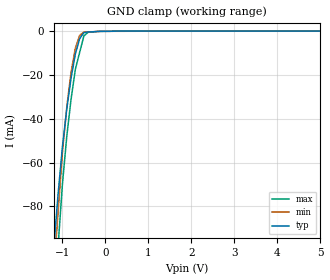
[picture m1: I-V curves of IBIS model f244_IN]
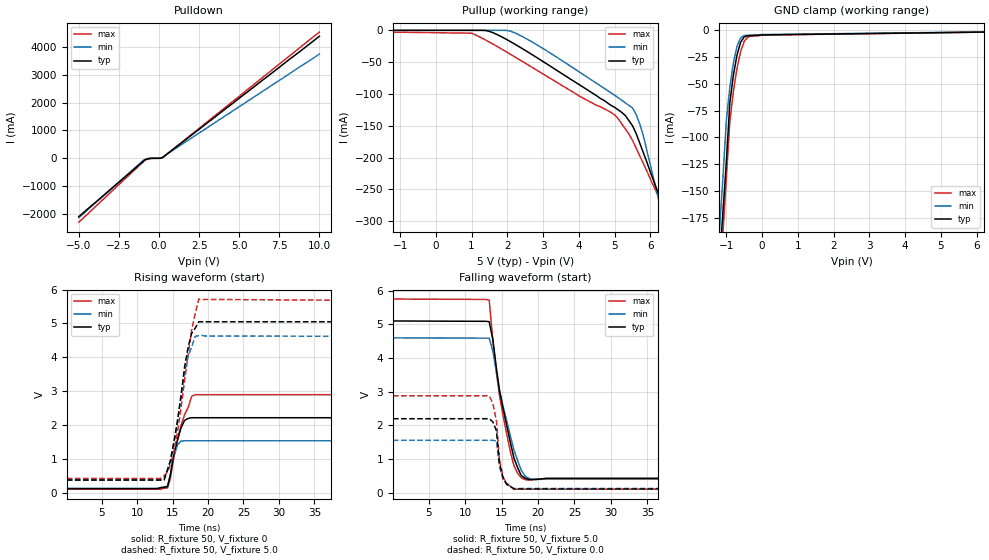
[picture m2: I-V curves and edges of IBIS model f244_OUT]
| TEXAS INSTRUMENTS INCORPORATED
| Standard Linear and Logic Group
| IBIS Model of SN74F244
| OCTAL BUFFERS/DRIVERS WITH 3-STATE OUTPUTS
| SOIC 20-pin (DW), SOP 20-pin (NS), SSOP 20-pin (DB), PDIP 20-pin (N)
[IBIS Ver]   3.2
[Comment Char]  |_char
[File Name]   sn74f244.ibs
[File Rev]   2.1 I_die
[Date]   Nov. 04, 2004
[Source]   File originated at Texas Instruments, Inc.
[Notes]   The following is a sample IBIS file for the F244.
   - FILE REV HISTORY
   - 2.1 Re-Release IBIS file on 11/05/04
   - Power-clamp data deleted as there is no power-clamp diode.
|   - All test data contained in this file are derived from
|   actual measurements.
|   - File created by Nobuhisa Ohtsubo, SLL Product Engineering.
[Disclaimer] Property of Texas Instruments Incorporated.  Unauthorized
   reproduction and/or distribution is strictly prohibited.
   This product is protected under copyright law.
   Created 2000, (C) Copyright 2000, Texas Instruments Inc.,
   All Rights Reserved.
   UNLESS THERE IS A SIGNED, WRITTEN AGREEMENT TO THE
   CONTRARY, TEXAS INSTRUMENTS () IS PROVIDING THE IBIS
   MODELS  AND WITHOUT ANY WARRANTY, EXPRESSED OR
   IMPLIED.  TI assumes no liability for:
   1) the accuracy of the IBIS models provided to your
   company;
   2) the proper functioning of these IBIS Models in your
   design or for any resulting applications; or
   3) infringement of patents, copyrights or intellectual
   property rights resulting from your use of these IBIS
   models.
   TI provides IBIS Models as a service to our customers.
   You and your company shall not distribute, sell or give
   these models to anyone else without prior written
   permission from TI.
   TI reserves the right to make changes to our products or
   to discontinue any semiconductor product or service
   without notice, and advises our customers to obtain the
   latest version of relevant information to verify, before
   placing orders, that the information being relied on is
   current.
   Please be aware that your receipt and use of the IBIS
   information provided shall serve as acceptance of these
   terms and conditions.  If you do not accept these terms,
   you should return or destroy the IBIS models and any
   other accompanying information immediately.
|   Component F244_DW
[Component]   f244_DW
[Manufacturer]  Texas Instruments, Inc.
[Package]
|   typ   min   max
R_pkg   0.038   0.033   0.045
L_pkg   5.012nH   4.110nH   6.349nH
C_pkg   0.717pF   0.530pF   0.868pF
[Pin]   signal_name   model_name   R_pin   L_pin   C_pin
1   1OE_NOT   f244_IN   0.058   5.115nH   0.725pF
2   1A1   f244_IN   0.053   4.591nH   0.724pF
3   2Y4   f244_OUT   0.049   3.754nH   0.572pF
4   1A2   f244_IN   0.029   2.549nH   0.388pF
5   2Y3   f244_OUT   0.031   2.317nH   0.316pF
6   1A3   f244_IN   0.031   2.317nH   0.316pF
7   2Y2   f244_OUT   0.029   2.556nH   0.399pF
8   1A4   f244_IN   0.049   3.754nH   0.579pF
9   2Y1   f244_OUT   0.053   4.591nH   0.724pF
10   GND   GND   0.058   5.115nH   0.725pF
11   2A1   f244_IN   0.058   5.115nH   0.725pF
12   1Y4   f244_OUT   0.053   4.591nH   0.724pF
13   2A2   f244_IN   0.049   3.754nH   0.579pF
14   1Y3   f244_OUT   0.029   2.557nH   0.399pF
15   2A3   f244_IN   0.031   2.317nH   0.316pF
16   1Y2   f244_OUT   0.031   2.317nH   0.316pF
17   2A4   f244_IN   0.029   2.557nH   0.399pF
18   1Y1   f244_OUT   0.049   3.754nH   0.579pF
19   2OE_NOT   f244_IN   0.053   4.591nH   0.724pF
20   VCC   POWER   0.058   5.115nH   0.725pF
|   Component F244_NS
[Component]   f244_NS
[Manufacturer]  Texas Instruments, Inc.
[Package]
|   typ   min   max
R_pkg   0.044   0.029   0.058
L_pkg   3.666nH   2.317nH   5.115nH
C_pkg   0.548pF   0.316pF   0.725pF
[Pin]   signal_name   model_name   R_pin   L_pin   C_pin
1   1OE_NOT   f244_IN   0.058   5.115nH   0.725pF
2   1A1   f244_IN   0.053   4.591nH   0.724pF
3   2Y4   f244_OUT   0.049   3.754nH   0.572pF
4   1A2   f244_IN   0.029   2.549nH   0.388pF
5   2Y3   f244_OUT   0.031   2.317nH   0.316pF
6   1A3   f244_IN   0.031   2.317nH   0.316pF
7   2Y2   f244_OUT   0.029   2.556nH   0.399pF
8   1A4   f244_IN   0.049   3.754nH   0.579pF
9   2Y1   f244_OUT   0.053   4.591nH   0.724pF
10   GND   GND   0.058   5.115nH   0.725pF
11   2A1   f244_IN   0.058   5.115nH   0.725pF
12   1Y4   f244_OUT   0.053   4.591nH   0.724pF
13   2A2   f244_IN   0.049   3.754nH   0.579pF
14   1Y3   f244_OUT   0.029   2.557nH   0.399pF
15   2A3   f244_IN   0.031   2.317nH   0.316pF
16   1Y2   f244_OUT   0.031   2.317nH   0.316pF
17   2A4   f244_IN   0.029   2.557nH   0.399pF
18   1Y1   f244_OUT   0.049   3.754nH   0.579pF
19   2OE_NOT   f244_IN   0.053   4.591nH   0.724pF
20   VCC   POWER   0.058   5.115nH   0.725pF
|   Component F244_DB
[Component]   f244_DB
[Manufacturer]  Texas Instruments, Inc.
[Package]
|   typ   min   max
R_pkg   0.040   0.035   0.051
L_pkg   3.495nH   3.035nH   4.314nH
C_pkg   0.420pF   0.346pF   0.502pF
[Pin]   signal_name   model_name   R_pin   L_pin   C_pin
1   1OE_NOT   f244_IN   0.049   4.310nH   0.502pF
2   1A1   f244_IN   0.048   3.903nH   0.487pF
3   2Y4   f244_OUT   0.035   3.189nH   0.396pF
4   1A2   f244_IN   0.035   3.036nH   0.347pF
5   2Y3   f244_OUT   0.035   3.035nH   0.367pF
6   1A3   f244_IN   0.035   3.035nH   0.367pF
7   2Y2   f244_OUT   0.035   3.036nH   0.347pF
8   1A4   f244_IN   0.035   3.189nH   0.397pF
9   2Y1   f244_OUT   0.047   3.899nH   0.488pF
10   GND   GND   0.051   4.314nH   0.500pF
11   2A1   f244_IN   0.051   4.314nH   0.500pF
12   1Y4   f244_OUT   0.047   3.899nH   0.488pF
13   2A2   f244_IN   0.035   3.189nH   0.397pF
14   1Y3   f244_OUT   0.035   3.036nH   0.346pF
15   2A3   f244_IN   0.035   3.035nH   0.367pF
16   1Y2   f244_OUT   0.035   3.035nH   0.367pF
17   2A4   f244_IN   0.035   3.036nH   0.346pF
18   1Y1   f244_OUT   0.035   3.189nH   0.397pF
19   2OE_NOT   f244_IN   0.047   3.899nH   0.488pF
20   VCC   POWER   0.051   4.314nH   0.502pF
|   Component F244_N
[Component]   f244_N
[Manufacturer]   Texas Instruments, Inc.
[Package]
|   typ   min   max
R_pkg   4.300e-02   3.800e-02   5.000e-02
L_pkg   7.384e-09   4.680e-09   1.032e-08
C_pkg   5.100e-13   2.310e-13   8.210e-13
[PIN]   signal_name   model_name   R_pin   L_pin   C_pin
1   1OE_NOT   f244_IN   4.200e-02   9.427e-09   8.100e-13
2   1A1   f244_IN   4.600e-02   8.544e-09   4.560e-13
3   2Y4   f244_OUT   4.800e-02   7.163e-09   4.350e-13
4   1A2   f244_IN   4.000e-02   4.825e-09   2.610e-13
5   2Y3   f244_OUT   4.000e-02   5.284e-09   6.480e-13
6   1A3   f244_IN   4.000e-02   4.686e-09   2.320e-13
7   2Y2   f244_OUT   4.000e-02   6.359e-09   4.890e-13
8   1A4   f244_IN   3.800e-02   7.982e-09   4.750e-13
9   2Y1   f244_OUT   4.300e-02   9.403e-09   4.750e-13
10   GND   GND   5.000e-02   1.032e-08   8.050e-13
11   2A1   f244_IN   5.000e-02   1.028e-08   8.100e-13
12   1Y4   f244_OUT   4.300e-02   9.383e-09   4.770e-13
13   2A2   f244_IN   3.800e-02   7.978e-09   4.760e-13
14   1Y3   f244_OUT   4.000e-02   6.302e-09   4.920e-13
15   2A3   f244_IN   4.000e-02   4.680e-09   2.310e-13
16   1Y2   f244_OUT   4.000e-02   5.284e-09   6.480e-13
17   2A4   f244_IN   4.000e-02   4.822e-09   2.610e-13
18   1Y1   f244_OUT   4.700e-02   7.118e-09   4.390e-13
19   2OE_NOT   f244_IN   4.600e-02   8.492e-09   4.610e-13
20   VCC   POWER   4.300e-02   9.348e-09   8.210e-13
| Models and submodels in the file (2): f244_IN (Input), f244_OUT (3-state)
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|   Model F244_IN
[Model]   f244_IN
Model_type  Input
Polarity   Inverting
Vinl = 0.8
Vinh = 2.0
| variable   typ   min   max
C_comp   1.33pf   1.00pf   1.66pf
[Temperature Range]   25   0   70
[Voltage Range]   5.0   4.75   5.25
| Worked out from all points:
|   GND clamp passes 1 mA (typ) near -0.51 V on its own axis
[GND Clamp]
|   Voltage   I(typ)   I(min)   I(max)
-5V       -1.09A     -1.45A     -1.18A
-1.2V     -98.7mA    -110mA     -123mA
-1.1V     -74.2mA    -82.4mA    -98mA
-1V       -52.8mA    -55.3mA    -69.8mA
-900mV    -35.7mA    -34.9mA    -48.3mA
-800mV    -21.6mA    -18.9mA    -31.2mA
-700mV    -10.5mA    -7.81mA    -17.5mA
-600mV    -3.51mA    -1.95mA    -9.77mA
-500mV    -712uA     -440uA     -2.16mA
-400mV    -387uA     -353uA     -532uA
-100mV    -112uA     -108uA     -114uA
5V        18.3nA     28.8pA     506pA
|   Model F244_OUT
[Model]   f244_OUT
Model_type  3-state
Polarity   Non-Inverting
Enable   Active-Low
Vmeas = 1.5v
Cref = 0pf
| variable   typ   min   max
C_comp   5.8pf   4.35pf   7.25pf
[Temperature Range]   25   0   70
[Voltage Range]   5.0   4.5   5.5
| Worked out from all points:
|   slope of the pulldown table from 0 to 0.75 V, typ, clamps not added: 2.84 ohm
|   rising waveform, R_fixture 50, V_fixture 0: 20-80 % time 1.33ns typ, 907ps min, 1.89ns max; typ from 0.125 V to 2.22 V
|   falling waveform, R_fixture 50, V_fixture 5.0: 20-80 % time 2.32ns typ, 2.58ns min, 2.23ns max; typ from 5.1 V to 0.433 V
|   rising waveform, R_fixture 50, V_fixture 5.0: 20-80 % time 2.01ns typ, 1.97ns min, 2.16ns max; typ from 0.383 V to 5.05 V
|   falling waveform, R_fixture 50, V_fixture 0.0: 20-80 % time 780ps typ, 750ps min, 899ps max; typ from 2.2 V to 0.116 V
[Pulldown]
|   Voltage   I(typ)   I(min)   I(max)
-5V       -2.1A      -2.14A     -2.3A
-1V       -124mA     -85mA      -139mA
-900mV    -67.6mA    -53.1mA    -85.1mA
-600mV    -11.3mA    -7.04mA    -20mA
200mV     17.1mA     11.5mA     22.1mA
500mV     149mA      147mA      144mA
10V       4.38A      3.74A      4.53A
[Pullup]
|   Voltage   II(typ)   I(min)   I(max)
-5V       68.9nA     2.4nA      202nA
1V        52.6nA     1.2nA      -4.5mA
1.5V      -1.67mA    1.2nA      -18.6mA
2.1V      -18.2mA    -1.56mA    -38.1mA
4.9V      -118mA     -98.4mA    -129mA
5.3V      -134mA     -114mA     -155mA
5.5V      -150mA     -122mA     -173mA
5.8V      -192mA     -165mA     -209mA
6.4V      -283mA     -306mA     -282mA
6.5V      -299mA     -329mA     -295mA
6.6V      -314mA     -353mA     -307mA
10V       -831mA     -1.15A     -722mA
[GND Clamp]
|   Voltage   I(typ)   I(min)   I(max)
-5V       -2.1A      -2.14A     -2.3A
-1.2V     -222mA     -192mA     -247mA
-1.1V     -173mA     -141mA     -193mA
-1V       -124mA     -85mA      -139mA
-900mV    -67.6mA    -53.1mA    -85.1mA
-800mV    -41.7mA    -30.2mA    -56.8mA
-700mV    -23.1mA    -14.9mA    -35.5mA
-600mV    -11.3mA    -7.04mA    -20mA
-500mV    -6.09mA    -4.84mA    -10.4mA
-400mV    -5.09mA    -4.57mA    -6.3mA
0V        -4.28mA    -3.91mA    -4.4mA
10V       12.8uA     19.1uA     11uA
[Ramp]
| variable   typ   min   max
dV/dt_r   1.230/1.267n   1.014/1.219n   1.428/1.413n
dV/dt_f   2.838/2.401n   2.532/2.618n   3.000/2.237n
R_load = 50
[Rising Waveform]
R_fixture = 50
V_fixture = 0
|   Time   V(typ)   V(min)   V(max)
97.7ps    125mV      136mV      114mV
14.3ns    186mV      201mV      154mV
14.7ns    540mV      537mV      430mV
15.2ns    1.17V      1.08V      1.08V
15.7ns    1.56V      1.42V      1.56V
16.2ns    1.92V      1.53V      1.99V
16.7ns    2.14V      1.54V      2.31V
17.7ns    2.22V      1.54V      2.85V
18.2ns    2.22V      1.54V      2.9V
49.8ns    2.22V      1.54V      2.9V
[Falling Waveform]
R_fixture = 50
V_fixture = 5.0
V_fixture_min = 4.5
V_fixture_max = 5.5
|   Time   V(typ)   V(min)   V(max)
97.7ps    5.1V       4.6V       5.75V
13.3ns    5.08V      4.59V      5.72V
13.8ns    4.55V      4.21V      4.53V
14.3ns    3.68V      3.56V      3.56V
14.7ns    3.06V      3.04V      2.91V
15.2ns    2.51V      2.57V      2.29V
16.7ns    1.03V      1.27V      802mV
17.7ns    514mV      667mV      448mV
19.6ns    396mV      401mV      410mV
49.8ns    433mV      421mV      410mV
[Rising Waveform]
R_fixture = 50
V_fixture = 5.0
V_fixture_min = 4.5
V_fixture_max = 5.5
|   Time   V(typ)   V(min)   V(max)
97.7ps    383mV      380mV      430mV
13.8ns    386mV      383mV      500mV
14.3ns    690mV      676mV      619mV
14.7ns    938mV      977mV      830mV
15.7ns    2.12V      2.11V      1.81V
16.7ns    3.71V      3.57V      3.32V
17.2ns    4.3V       4.03V      4.07V
17.7ns    4.71V      4.31V      4.81V
18.7ns    5.05V      4.64V      5.72V
49.8ns    5.05V      4.62V      5.67V
[Falling Waveform]
R_fixture = 50
V_fixture = 0.0
|   Time   V(typ)   V(min)   V(max)
97.7ps    2.2V       1.56V      2.88V
13.3ns    2.2V       1.56V      2.88V
13.8ns    2.11V      1.56V      2.66V
14.3ns    1.84V      1.54V      2.13V
14.7ns    890mV      789mV      993mV
15.2ns    448mV      411mV      469mV
15.7ns    265mV      242mV      283mV
16.7ns    116mV      132mV      110mV
49.8ns    116mV      132mV      110mV
